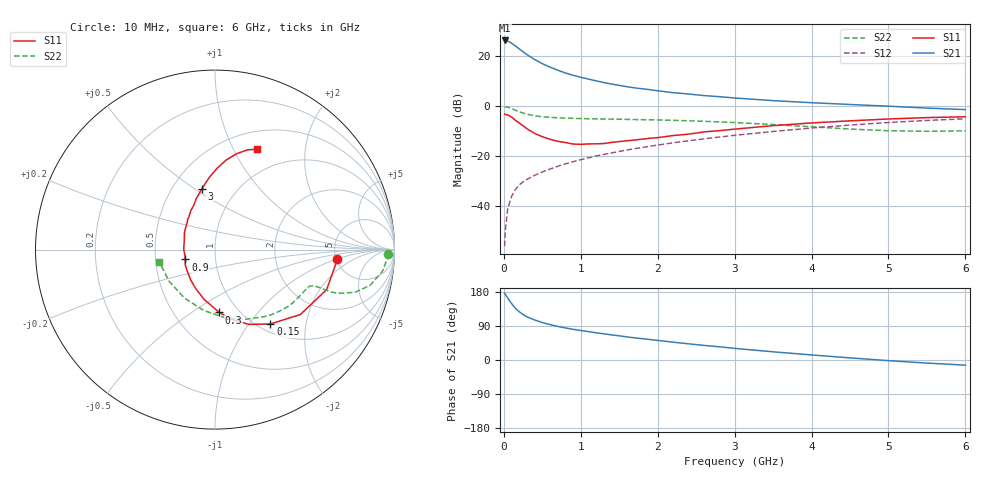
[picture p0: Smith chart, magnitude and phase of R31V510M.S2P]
! SIEMENS Small Signal Semiconductors
! BFR181
! Si NPN RF Bipolar Junction Transistor in SOT23
! VCE = 1.5 V  IC = 10 mA
! Common Emitter S-Parameters:  May  1996
# GHz  S  MA  R  50
!  f  S11  S21  S12  S22
! GHz  MAG  ANG  MAG  ANG  MAG  ANG  MAG  ANG
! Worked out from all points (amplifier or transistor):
!   36 points, 10 MHz to 6 GHz, reference 50 ohm
!   highest |S21| = 26.1 dB at 10 MHz (marker M1)
!   |S21| within 3 dB of that: start of sweep to 185 MHz
!   unconditionally stable (mu >= 1): 541 MHz to 2.929 GHz
!   at 250 MHz: K = 0.68, MSG = 25.9 dB, |S12| = -30.3 dB
!   at 1.4 GHz: K = 1.14, MAG = 11.5 dB, |S12| = -18.8 dB
!   at 6 GHz: K = 0.90, MSG = 1.8 dB, |S12| = -5.1 dB
!   S11 on the Smith chart (normalised r, x): 10 MHz: 5.14, -0.97; 150 MHz: 1.13, -1.28; 300 MHz: 0.81, -0.65; 900 MHz: 0.71, -0.08; 3 GHz: 0.69, +0.53; 6 GHz: 0.70, +1.25
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0.01  0.6842 -4.2  20.11 176.6  0.0016 88.9  0.9642 -1.3
0.02  0.6746 -8.1  19.96 173.0  0.0034 80.9  0.9603 -3.1
0.05  0.6608 -19.7  19.6 163.5  0.0089 78.8  0.9417 -7.3
0.1  0.5978 -37.2  17.78 149.2  0.0156 74.9  0.8866 -13.0
0.15  0.5168 -53.3  15.65 136.4  0.0216 68.9  0.818 -16.8
0.2  0.4572 -65.7  13.67 127.4  0.0266 67.0  0.7616 -18.6
0.25  0.401 -76.2  11.95 120.0  0.0306 64.8  0.7191 -19.7
0.3  0.3507 -86.2  10.5 114.0  0.0342 65.1  0.6828 -20.1
0.4  0.2832 -102.5  8.408 105.7  0.0413 65.5  0.6358 -20.0
0.5  0.2428 -116.1  6.933 98.7  0.0482 66.4  0.6085 -20.0
0.6  0.2162 -128.9  5.918 93.4  0.0551 67.3  0.5908 -20.1
0.7  0.1967 -141.5  5.147 88.7  0.0624 68.5  0.5788 -20.4
0.9  0.1735 -161.6  4.068 81.0  0.0773 69.1  0.5634 -21.4
1.1  0.1744 179.4  3.414 74.9  0.0921 69.8  0.5543 -23.2
1.3  0.1777 164.1  2.914 69.1  0.1078 69.7  0.5469 -25.3
1.6  0.2015 145.2  2.407 60.9  0.1319 68.9  0.5377 -29.0
2.2  0.256 121.6  1.832 47.1  0.1838 66.0  0.5148 -38.1
3  0.3441 102.6  1.436 30.7  0.2587 59.8  0.4654 -53.2
3.5  0.4038 94.5  1.272 21.6  0.3091 54.9  0.4252 -65.9
4.5  0.5035 82.8  1.066 5.6  0.4147 42.8  0.3448 -100.6
5.5  0.5835 72.1  0.903 -8.1  0.5124 28.7  0.311 -145.3
6  0.6069 67.2  0.843 -13.6  0.553 21.1  0.3183 -167.8
